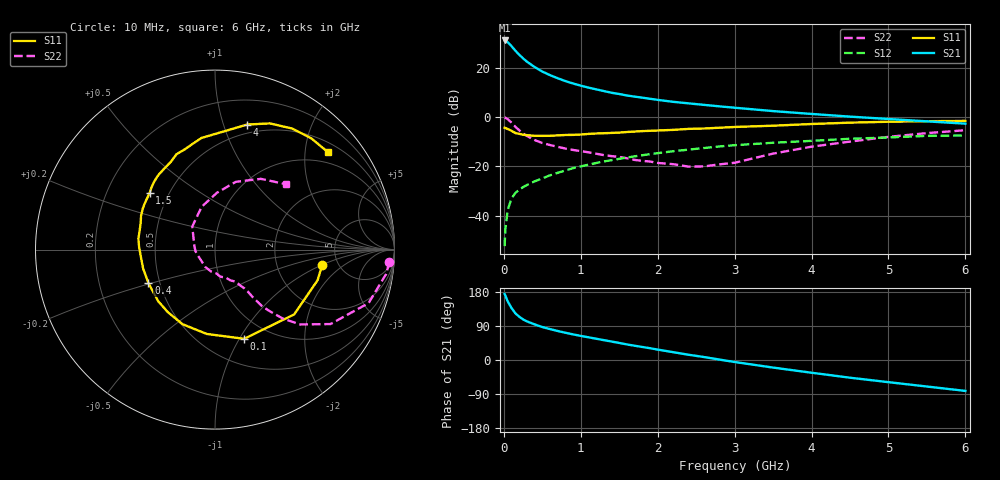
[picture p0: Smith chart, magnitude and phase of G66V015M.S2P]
! SIEMENS Small Signal Semiconductors
! BFG193
! Si NPN RF Bipolar Junction Transistor in SOT223
! VCE = 6 V  IC = 15 mA
! Common Emitter S-Parameters:  August  1996
# GHz  S  MA  R  50
!  f  S11  S21  S12  S22
! GHz  MAG  ANG  MAG  ANG  MAG  ANG  MAG  ANG
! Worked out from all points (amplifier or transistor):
!   36 points, 10 MHz to 6 GHz, reference 50 ohm
!   highest |S21| = 31.0 dB at 10 MHz (marker M1)
!   |S21| within 3 dB of that: start of sweep to 118.6 MHz
!   unconditionally stable (mu >= 1): 782.4 MHz to 2.39 GHz
!   at 250 MHz: K = 0.65, MSG = 26.1 dB, |S12| = -28.5 dB
!   at 1.4 GHz: K = 1.06, MAG = 12.2 dB, |S12| = -17.5 dB
!   at 6 GHz: K = 0.87, MSG = 2.4 dB, |S12| = -7.5 dB
!   S11 on the Smith chart (normalised r, x): 10 MHz: 3.75, -1.01; 100 MHz: 0.77, -1.05; 400 MHz: 0.43, -0.19; 1.5 GHz: 0.39, +0.32; 4 GHz: 0.42, +1.20; 6 GHz: 0.72, +2.52
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0.01  0.6032 -8.2  35.57 174.2  0.0024 91.8  0.9745 -4.0
0.02  0.5966 -16.6  35.13 169.8  0.0053 84.6  0.9634 -8.1
0.05  0.57 -39.3  32.72 154.7  0.013 73.4  0.9061 -19.2
0.1  0.5228 -71.9  27.28 137.1  0.0224 64.2  0.7657 -32.8
0.15  0.4722 -95.6  22 123.1  0.0288 58.7  0.6319 -41.3
0.2  0.4534 -113.5  18.3 114.3  0.0336 56.5  0.5381 -45.5
0.25  0.4364 -127.1  15.39 107.2  0.0378 55.7  0.4612 -48.3
0.3  0.4276 -137.8  13.23 101.9  0.0417 55.5  0.4124 -50.2
0.4  0.415 -153.3  10.29 94.0  0.0494 56.2  0.3405 -51.5
0.5  0.414 -165.1  8.328 87.0  0.0568 56.5  0.2962 -52.0
0.6  0.4149 -174.3  7.044 81.6  0.0656 57.3  0.2696 -52.9
0.7  0.423 178.2  6.091 76.5  0.0737 57.0  0.2481 -54.6
0.9  0.4331 165.5  4.768 67.6  0.0917 55.5  0.2142 -57.0
1.1  0.4529 155.5  3.932 59.9  0.1077 53.8  0.1921 -63.3
1.5  0.482 139.0  2.918 45.0  0.1416 47.6  0.1545 -78.1
2.2  0.5471 116.8  2.028 20.7  0.2016 34.6  0.1104 -120.1
2.8  0.6041 101.5  1.641 1.2  0.2519 22.0  0.1092 -175.3
3.5  0.6649 84.7  1.315 -20.0  0.2999 5.6  0.1806 134.5
4  0.7193 75.6  1.151 -33.6  0.3277 -4.0  0.2496 107.4
4.5  0.7667 66.5  1.016 -46.7  0.3615 -14.1  0.3167 88.1
5.5  0.8199 49.1  0.815 -70.0  0.4132 -37.9  0.47 57.0
6  0.8313 40.7  0.731 -81.6  0.4212 -51.7  0.5387 42.5
